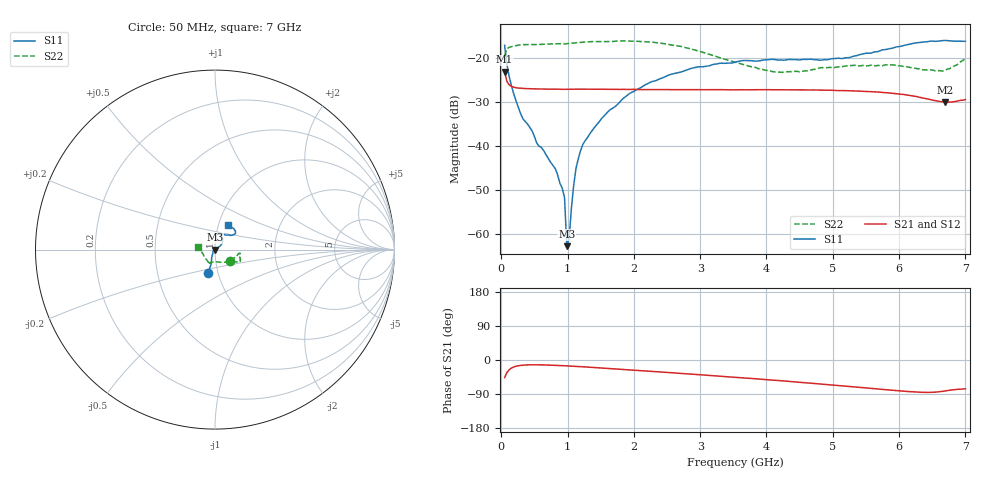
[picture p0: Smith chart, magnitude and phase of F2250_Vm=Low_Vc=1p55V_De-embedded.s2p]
! Integrated Device Technology
! Corporate Headquarters
! 6024 Silver Creek Valley Road
! San Jose, CA 95138  USA
! Phone:  1-408-284-8200
! Toll Free:  1-800-223-1366
! Webpage:  http://www.idt.com/
! Timing and RF Division
! 515 Groton Road, Suite 102
! Westford, MA 01886-6024
! Device:  F2250
! Description: Voltage Variable RF Attenuator
! Frequency:  50.0 -  6000.00 MHz
! Package:  3x3 mm Thin QFN Plastic Package: 16 pin
! Ports:  2 RF, 3 DC
!  Pin  1  = GND
!  Pin  2  = NC
!  Pin  3  = RF1  = Port 1
!  Pin  4  = NC
!  Pin  5  = GND
!  Pin  6  = GND
!  Pin  7  = GND
!  Pin  8  = GND
!  Pin  9  = NC
!  Pin 10  = RF2  = Port 2
!  Pin 11  = NC
!  Pin 12  = GND
!  Pin 13  = GND
!  Pin 14  = VCNTRL
!  Pin 15  = VDD
!  Pin 16  = VMODE
! Vcntrl:  1.550 Volts
! Vmode:  +0.000 Volts
! Vdd:  +3.30  Volts
! Current:  1.190 mA
! Data:  The device was measured on a the F2250 evaluation board which has
!  individual transmission lines to the RF pins.  Data was collected
!  using a calibrated network analyzer.  The evaluation board was
!  de-embedded using a TRL calibration technique.
!  The reference plane is the edge of the package pin.
! Misc:  SN 10
!  Action Tracker AT0258
! Date Measured:  2014-11-26
! Date:  2015-10-15  MJV
! Note:
!  Integrated Device Technology supplies this data as a sample of measured
!  data at the package pin for this product.  Your particular data for this
!  product may vary.
!  Data was taken at 25 degrees C.
!  Integrated Device Technology reserves the right to change this data at anytime.
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# GHz S dB R 50
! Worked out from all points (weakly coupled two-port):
!   201 points, 50 MHz to 7 GHz, reference 50 ohm
!   highest |S21| = -23.17 dB at 50 MHz (marker M1); lowest = -30.1 dB at 6.687 GHz (marker M2)
!   lowest |S11| = -62.7 dB at 988.2 MHz (marker M3), VSWR 1.00, Z = 49.9 + j0.0281 ohm
!   |S11| at or under -10 dB: start of sweep to end of sweep
!   |S22| runs from -23.3 to -16.2 dB; largest |S21 - S12| = 0.00024
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0.05  -17.19 -106.8  -23.17 -46.2  -23.16 -46.2  -19.57 -35.5
0.1195  -24.30 -108.6  -26.15 -25.5  -26.16 -25.5  -17.65 -11.4
0.29325  -32.75 -120.5  -26.90 -14.2  -26.90 -14.2  -17.06 -8.8
0.5365  -39.37 -144.8  -27.07 -12.7  -27.08 -12.7  -17.02 -10.3
0.8145  -45.11 177.7  -27.12 -14.1  -27.11 -14.1  -16.87 -14.7
0.91875  -49.53 154.0  -27.16 -14.9  -27.11 -14.9  -16.83 -16.7
0.9535  -51.60 -179.3  -27.15 -15.2  -27.11 -15.2  -16.89 -16.9
0.98825  -62.67 157.5  -27.13 -15.5  -27.12 -15.5  -16.82 -17.3
1.023  -60.95 54.3  -27.14 -15.8  -27.13 -15.8  -16.76 -17.4
1.05775  -54.00 40.4  -27.14 -16.1  -27.14 -16.1  -16.73 -17.7
1.12725  -45.00 29.9  -27.12 -16.8  -27.11 -16.8  -16.62 -18.9
1.2315  -39.59 27.7  -27.12 -17.9  -27.10 -17.9  -16.47 -20.6
1.5095  -33.84 31.5  -27.15 -21.1  -27.12 -21.1  -16.36 -22.7
1.82225  -29.46 34.3  -27.17 -24.7  -27.15 -24.7  -16.21 -25.1
2.37825  -24.87 44.2  -27.21 -31.3  -27.21 -31.3  -16.64 -28.4
2.93425  -22.17 57.8  -27.24 -38.1  -27.22 -38.2  -18.33 -34.2
3.525  -21.02 71.0  -27.28 -45.6  -27.26 -45.7  -21.01 -52.8
4.11575  -20.39 78.7  -27.26 -53.4  -27.24 -53.4  -23.20 -80.8
4.7065  -20.43 71.5  -27.30 -61.8  -27.30 -61.8  -22.66 -104.5
5.85325  -17.96 39.6  -27.98 -79.2  -27.98 -79.3  -21.68 -114.0
6.68725  -16.10 48.2  -30.08 -81.9  -30.09 -81.9  -22.85 -163.4
7  -16.28 62.8  -29.47 -75.9  -29.48 -75.9  -20.26 172.3
